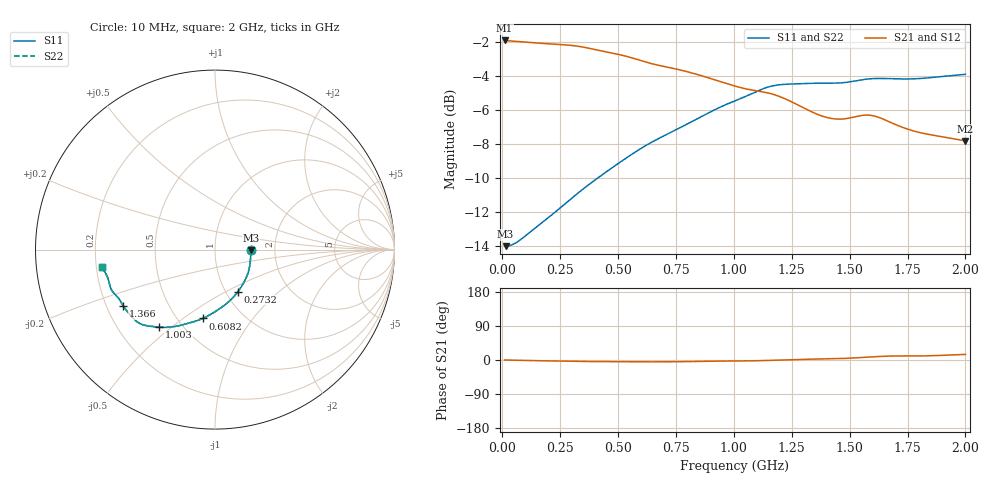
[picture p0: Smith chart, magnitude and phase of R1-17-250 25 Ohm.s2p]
!version-1
!date-02.2021
!Series
#	GHZ	S	RI	R	50.0
!	FREQ.GHZ	S11RE	S11IM	S21RE	S21IM	S12RE	S12IM	S22RE	S22IM
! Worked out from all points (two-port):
!   500 points, 10 MHz to 2 GHz, reference 50 ohm
!   highest |S21| = -1.94 dB at 10 MHz (marker M1); lowest = -7.8 dB at 2 GHz (marker M2)
!   |S21| within 3 dB of the highest: start of sweep to 1.121 GHz
!   lowest |S11| = -14.0 dB at 13.99 MHz (marker M3), VSWR 1.50, Z = 75 - j0.666 ohm
!   |S11| at or under -10 dB: start of sweep to 411.4 MHz
!   |S22| runs from -14.0 to -3.9 dB; largest |S21 - S12| = 0
!   S11 on the Smith chart (normalised r, x): 10 MHz: 1.50, -0.00; 273.2 MHz: 1.14, -0.57; 608.2 MHz: 0.66, -0.60; 1.003 GHz: 0.38, -0.45; 1.366 GHz: 0.27, -0.26; 2 GHz: 0.22, -0.07
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0.01  0.2 -7.3e-05  0.8 -3.7e-05  0.8 -3.7e-05  0.2 -7.3e-05
0.013988  0.1999 -0.00426  0.7996 -0.000824  0.7996 -0.000824  0.1999 -0.00426
0.0578557  0.1981 -0.05  0.7951 -0.00937  0.7951 -0.00937  0.1981 -0.05
0.133627  0.186 -0.124  0.7876 -0.0224  0.7876 -0.0224  0.186 -0.124
0.273206  0.1279 -0.2343  0.7752 -0.0432  0.7752 -0.0432  0.1279 -0.2343
0.34499  0.0891 -0.2786  0.7642 -0.0515  0.7642 -0.0515  0.0891 -0.2786
0.464629  0.0172 -0.3353  0.7346 -0.0571  0.7346 -0.0571  0.0172 -0.3353
0.608196  -0.0684 -0.3837  0.6926 -0.0598  0.6926 -0.0598  -0.0684 -0.3837
0.675992  -0.1085 -0.3988  0.6739 -0.0574  0.6739 -0.0574  -0.1085 -0.3988
0.875391  -0.2266 -0.4289  0.6252 -0.0381  0.6252 -0.0381  -0.2266 -0.4289
1.00301  -0.31 -0.4322  0.5882 -0.0271  0.5882 -0.0271  -0.31 -0.4322
1.00699  -0.3126 -0.432  0.5871 -0.0269  0.5871 -0.0269  -0.3126 -0.432
1.10271  -0.379 -0.4243  0.5688 -0.019  0.5688 -0.019  -0.379 -0.4243
1.15455  -0.4157 -0.4133  0.56 -0.0103  0.56 -0.0103  -0.4157 -0.4133
1.24627  -0.4684 -0.3691  0.5303 0.00738  0.5303 0.00738  -0.4684 -0.3691
1.338  -0.5038 -0.3246  0.4935 0.0198  0.4935 0.0198  -0.5038 -0.3246
1.36591  -0.5117 -0.3129  0.4843 0.0221  0.4843 0.0221  -0.5117 -0.3129
1.45365  -0.5324 -0.2776  0.4697 0.0298  0.4697 0.0298  -0.5324 -0.2776
1.58525  -0.5729 -0.2306  0.4789 0.0665  0.4789 0.0665  -0.5729 -0.2306
1.669  -0.5864 -0.1968  0.4557 0.0823  0.4557 0.0823  -0.5864 -0.1968
1.82054  -0.6033 -0.1434  0.4198 0.0802  0.4198 0.0802  -0.6033 -0.1434
2  -0.6291 -0.0984  0.3931 0.1037  0.3931 0.1037  -0.6291 -0.0984
